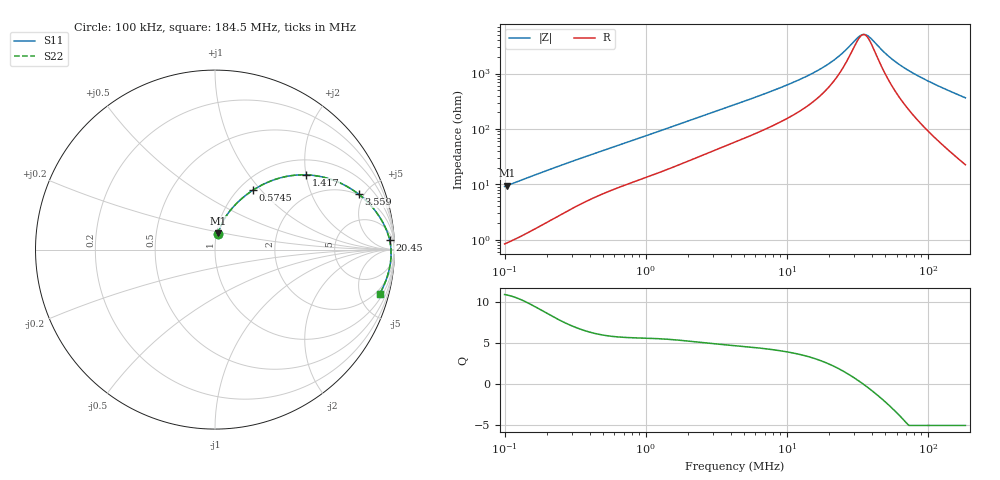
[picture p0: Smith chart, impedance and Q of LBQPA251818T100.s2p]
! LBQPA251818T100  S-PARAMETER MODEL  ( General Type )
! Model Generated by TAIYO YUDEN Corporation (http://www.ty-top.com)
! Version 1.0
! TAIYO YUDEN Control No. 191025NI43SB-FBB
! Copyright(c) 2019 TAIYO YUDEN CO.,LTD. All Rights Reserved.
! Product Description (link to TY-COMPAS)
! https://ds.yuden.co.jp/TYCOMPAS/or/detail?pn=LBQPA251818T100K&u=M
! Products Name : Inductors
! Characteristics :
!  Inductance : 10 uH , SRF(min) : 30 MHz , DC Resistance(max) : 0.468 Ohm
!  Rated Current : Saturation :480 mA , Temp Rise : 375 mA (20 degC)
!  Case Size : 2.5 x 1.8 / 0.098 x 0.071 [mm/inch] , Thickness : 1.8 / 0.071 [mm/inch]
!  (Conditions: Temperature = 25 degC , DC Bias Current/Voltage = 0A / 0V)
! External Node Assignments :
!  1  o---GGG---o  2
! GND o---------o GND
! Frequency Range : 0.1MHz  -  184.468258MHz  [ 402 STEP ]
# MHz S RI R 50
! Freq[MHz].  S11 Real  S11 Imag  S21 Real  S21 Imag  S12 Real  S12 Imag  S22 Real  S22 Imag
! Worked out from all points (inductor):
!   401 points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, 100 kHz to 184.5 MHz, reference 50 ohm
!   read as one part in series: L = 14.4 uH near 103.8 kHz
!   highest Q = 10.8 at 103.8 kHz (marker M1), where L = 14.4 uH
!   self-resonance near 34.89 MHz
!   S11 on the Smith chart (normalised r, x): 100 kHz: 1.02, +0.18; 574.5 kHz: 1.16, +0.91; 1.417 MHz: 1.37, +2.01; 3.559 MHz: 1.95, +4.55; 20.45 MHz: 13, +29; 184.5 MHz: 1.45, -7.29
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0.1  0.0163 0.0886  0.9837 -0.0886  0.9837 -0.0886  0.0163 0.0886
0.103832  0.0172 0.0918  0.9828 -0.0918  0.9828 -0.0918  0.0172 0.0918
0.204297  0.0505 0.1677  0.9495 -0.1677  0.9495 -0.1677  0.0505 0.1677
0.352405  0.1141 0.2511  0.8859 -0.2511  0.8859 -0.2511  0.1141 0.2511
0.574549  0.2119 0.3313  0.7881 -0.3313  0.7881 -0.3313  0.2119 0.3313
1.241892  0.4592 0.4157  0.5408 -0.4157  0.5408 -0.4157  0.4592 0.4157
1.416568  0.5091 0.4164  0.4909 -0.4164  0.4909 -0.4164  0.5091 0.4164
2.309523  0.6828 0.3776  0.3172 -0.3776  0.3172 -0.3776  0.6828 0.3776
3.558875  0.7996 0.3093  0.2004 -0.3093  0.2004 -0.3093  0.7996 0.3093
4.294977  0.8381 0.2764  0.1619 -0.2764  0.1619 -0.2764  0.8381 0.2764
8.941043  0.9318 0.1572  0.0682 -0.1572  0.0682 -0.1572  0.9318 0.1572
15.13571  0.9629 0.0888  0.0371 -0.0888  0.0371 -0.0888  0.9629 0.0888
20.44747  0.9728 0.0551  0.0272 -0.0551  0.0272 -0.0551  0.9728 0.0551
25.14504  0.9771 0.0334  0.0229 -0.0334  0.0229 -0.0334  0.9771 0.0334
32.10664  0.9801 0.00844  0.0199 -0.00844  0.0199 -0.00844  0.9801 0.00844
34.61418  0.9806 0.000804  0.0194 -0.000804  0.0194 -0.000804  0.9806 0.000804
36.62254  0.9809 -0.00495  0.0191 0.00495  0.0191 0.00495  0.9809 -0.00495
38.74743  0.9811 -0.0107  0.0189 0.0107  0.0189 0.0107  0.9811 -0.0107
53.33896  0.9803 -0.0449  0.0197 0.0449  0.0197 0.0449  0.9803 -0.0449
66.83781  0.9776 -0.0716  0.0224 0.0716  0.0224 0.0716  0.9776 -0.0716
86.96199  0.9714 -0.1069  0.0286 0.1069  0.0286 0.1069  0.9714 -0.1069
184.4683  0.917 -0.2466  0.083 0.2466  0.083 0.2466  0.917 -0.2466
